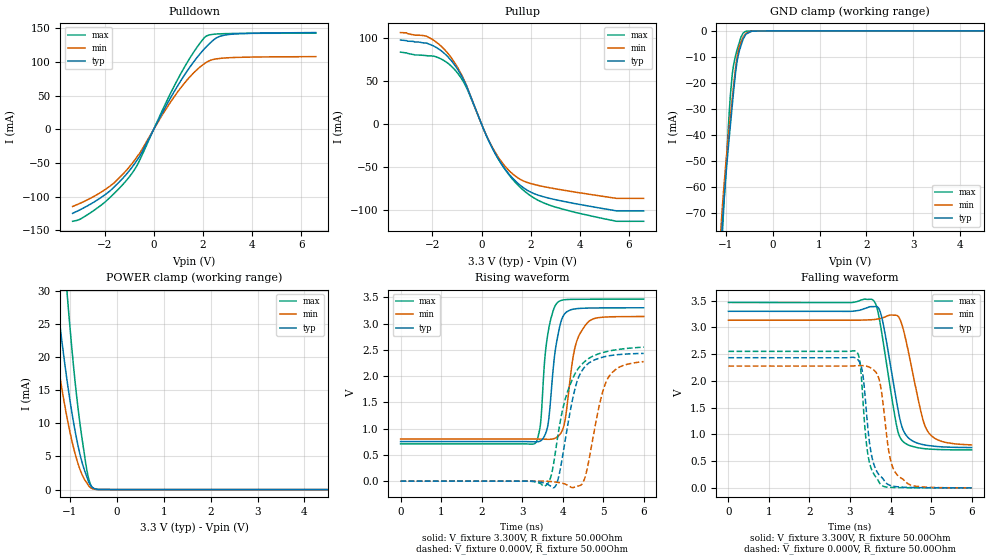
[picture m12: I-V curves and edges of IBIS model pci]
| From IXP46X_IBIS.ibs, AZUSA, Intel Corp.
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[Model]   pci
Model_type   I/O
Vinl = 950.000mV
Vinh = 1.500V
Vmeas = 1.500V
Cref = 0.000F
|   typ   min   max
C_comp   3.000pF   2.700pF   3.300pF
[Voltage Range]   3.300V   3.135V   3.465V
[Temperature Range]   25.0   110.0   -40.0
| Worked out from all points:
|   slope of the pulldown table from 0 to 0.495 V, typ, clamps not added: 14.5 ohm
|   slope of the pullup table from 0 to 0.495 V, typ, clamps not added: 16 ohm
|   GND clamp passes 1 mA (typ) near -0.54 V on its own axis
|   POWER clamp passes 1 mA (typ) near -0.59 V on its own axis
|   falling waveform, V_fixture 3.300V, R_fixture 50.00Ohm: 20-80 % time 352ps typ, 396ps min, 346ps max; typ from 3.3 V to 0.753 V
|   rising waveform, V_fixture 3.300V, R_fixture 50.00Ohm: 20-80 % time 218ps typ, 269ps min, 187ps max; typ from 0.753 V to 3.3 V
|   rising waveform, V_fixture 0.000V, R_fixture 50.00Ohm: 20-80 % time 377ps typ, 377ps min, 490ps max; typ from 0 V to 2.43 V
|   falling waveform, V_fixture 0.000V, R_fixture 50.00Ohm: 20-80 % time 227ps typ, 250ps min, 186ps max; typ from 2.43 V to 0 V
[Pulldown]
|   Voltage   I(typ)   I(min)   I(max)
-3.3V     -124.6mA   -114.4mA   -136.4mA
-2.99V    -119.2mA   -109.6mA   -133.2mA
-1.99V    -97.22mA   -89.65mA   -108.2mA
-1.605V   -85.39mA   -79.22mA   -94.97mA
-885mV    -56.4mA    -50.94mA   -65.35mA
-525mV    -37.09mA   -32.82mA   -42.22mA
940mV     62.44mA    53.71mA    71.6mA
1.535V    95.49mA    80.32mA    109.3mA
2.08V     120mA      97.84mA    136.7mA
2.545V    135.5mA    104.5mA    141.4mA
2.89V     139.8mA    105.8mA    141.9mA
6.595V    143.5mA    107.9mA    142.6mA
[GND Clamp]
|   Voltage   I(typ)   I(min)   I(max)
-3.3V     -1.837A    -1.782A    -2.142A
-1.11V    -85.01mA   -78.04mA   -93.41mA
-1.065V   -72.56mA   -66.27mA   -76.24mA
-1.06V    -71.11mA   -65.16mA   -74.6mA
-925mV    -41.22mA   -37.4mA    -31.6mA
-860mV    -28.8mA    -26.04mA   -16.75mA
-790mV    -16.27mA   -14.37mA   -9.57mA
-750mV    -11.01mA   -9.296mA   -6.861mA
-675mV    -5.754mA   -4.387mA   -2.478mA
-580mV    -1.626mA   -1.201mA   -252.6uA
0V        -56.89nA   -17.57nA   -32.79pA
6.595V    0A         0A         0A
[Pullup]
|   Voltage   I(typ)   I(min)   I(max)
-3.3V     98.13mA    106.8mA    83.99mA
-2.035V   92.21mA    99.32mA    79.58mA
-1.47V    81.33mA    85.81mA    73.06mA
-1.065V   67.76mA    70.28mA    62.68mA
-625mV    45.23mA    45.89mA    43.19mA
440mV     -28.01mA   -26.99mA   -27.96mA
910mV     -50.37mA   -47.38mA   -50.87mA
1.465V    -68.53mA   -62.27mA   -70.53mA
2.15V     -81.02mA   -70.21mA   -86.2mA
3.05V     -88.15mA   -75.43mA   -96.88mA
5.5V      -100.9mA   -86.34mA   -113mA
6.595V    -100.9mA   -86.34mA   -113mA
[POWER Clamp]
|   Voltage   I(typ)   I(min)   I(max)
-3.3V     221.1mA    178.3mA    345.2mA
-1.5V     44.33mA    31.93mA    76.54mA
-1.44V    39.94mA    28.54mA    69.34mA
-1.27V    28.47mA    19.76mA    50.25mA
-1.06V    16.5mA     10.87mA    29.8mA
-1.045V   15.76mA    10.32mA    28.49mA
-890mV    8.924mA    5.478mA    16.42mA
-770mV    4.917mA    2.796mA    9.212mA
-635mV    1.89mA     986.7uA    2.845mA
-570mV    776uA      354.8uA    984.2uA
-515mV    310.8uA    129.8uA    274uA
6.595V    0A         0A         0A
[Ramp]
R_load = 50.00Ohm
|   typ   min   max
dV/dt_r   1.459V/377.159ps   1.366V/375.703ps   1.531V/489.766ps
dV/dt_f   1.528V/351.414ps   1.400V/395.616ps   1.654V/345.636ps
[Falling Waveform]
V_fixture = 3.300V
V_fixture_min = 3.135V
V_fixture_max = 3.465V
R_fixture = 50.00Ohm
|   Time   V(typ)   V(min)   V(max)
0s        3.3V       3.135V     3.465V
3.57ns    3.387V     3.144V     3.508V
3.66ns    3.388V     3.152V     3.379V
3.78ns    3.197V     3.172V     2.912V
4.16ns    1.568V     3.222V     1.125V
4.38ns    988.5mV    2.757V     824.6mV
4.75ns    816.8mV    1.423V     740.7mV
4.9ns     794.6mV    1.077V     727.9mV
5.25ns    767.3mV    871.5mV    714.9mV
6ns       753.2mV    802.4mV    708.3mV
[Rising Waveform]
V_fixture = 3.300V
V_fixture_min = 3.135V
V_fixture_max = 3.465V
R_fixture = 50.00Ohm
|   Time   V(typ)   V(min)   V(max)
0s        753.2mV    802.4mV    708.3mV
3.31ns    748.7mV    802.6mV    714.2mV
3.45ns    765.1mV    799.9mV    1.062V
3.55ns    855.5mV    798.1mV    2.232V
3.63ns    1.039V     797mV      2.776V
3.85ns    2.639V     832.8mV    3.38V
4.05ns    3.185V     1.12V      3.453V
4.29ns    3.277V     2.492V     3.461V
4.56ns    3.293V     2.966V     3.463V
6ns       3.3V       3.135V     3.465V
[Rising Waveform]
V_fixture = 0.000V
V_fixture_min = 0.000V
V_fixture_max = 0.000V
R_fixture = 50.00Ohm
|   Time   V(typ)   V(min)   V(max)
0s        621.9nV    214.4nV    1.742nV
3.55ns    -36.59mV   104.3uV    -94.6mV
3.79ns    -122.4mV   -12.84mV   393.1mV
4.06ns    761.2mV    -54.78mV   1.549V
4.28ns    1.678V     -117.4mV   2.006V
4.44ns    2.053V     -78.29mV   2.195V
4.58ns    2.203V     149.2mV    2.3V
4.91ns    2.342V     1.458V     2.43V
5.1ns     2.38V      1.934V     2.469V
6ns       2.432V     2.276V     2.551V
[Falling Waveform]
V_fixture = 0.000V
V_fixture_min = 0.000V
V_fixture_max = 0.000V
R_fixture = 50.00Ohm
|   Time   V(typ)   V(min)   V(max)
0s        2.432V     2.276V     2.551V
3.14ns    2.427V     2.281V     2.555V
3.24ns    2.343V     2.285V     2.371V
3.31ns    2.149V     2.285V     1.742V
3.46ns    975.9mV    2.261V     543mV
3.58ns    460.3mV    2.208V     267.7mV
3.75ns    218.1mV    1.921V     69.77mV
3.97ns    51.23mV    627.7mV    10.43mV
4.16ns    20.69mV    245.8mV    5.326mV
6ns       621.9nV    214.4nV    1.742nV
